(* Logix 5000 AddOnInstructionDefinition export AMCI_MAM; software revision 20.05 *)

TYPE AMCI_Motion_Axis_Output_Data :
STRUCT
   Control_Word_0 : INT;
   Control_Word_1 : INT;
   Position_or_Distance : DINT;
   Programmed_Speed : DINT;
   Acceleration : INT;
   Deceleration : INT;
   Output_Word_8 : INT;
   Output_Word_9 : INT;
END_STRUCT
END_TYPE

TYPE AMCI_Motion_Axis_Input_Data :
STRUCT
   Moving_CW : BOOL;
   Moving_CCW : BOOL;
   In_Hold_State : BOOL;
   Stopped : BOOL;
   At_Home : BOOL;
   Accelerating : BOOL;
   Decelerating : BOOL;
   Move_Complete : BOOL;
   Status_Word_0_Bit_8 : BOOL;
   Status_Word_0_Bit_9 : BOOL;
   Position_Invalid : BOOL;
   Input_Error : BOOL;
   Command_Error : BOOL;
   Configuration_Error : BOOL;
   Module_OK : BOOL;
   Mode_Flag : BOOL;
   IN1_Active : BOOL;
   IN2_Active : BOOL;
   IN3_Active : BOOL;
   IN4_Active : BOOL;
   Status_Word_1_Bit_4 : BOOL;
   Status_Word_1_Bit_5 : BOOL;
   Connection_Was_Lost : BOOL;
   Driver_Fault : BOOL;
   Status_Word_1_Bit_8 : BOOL;
   Invalid_Jog_Change : BOOL;
   Status_Word_1_Bit_10 : BOOL;
   Heartbeat_Bit : BOOL;
   Status_Word_1_Bit_12 : BOOL;
   Status_Word_1_Bit_13 : BOOL;
   Stall_Detected : BOOL;
   Drive_Is_Enabled : BOOL;
   Motor_Position : DINT;
   Encoder_Position : DINT;
   Trapped_Encoder_Position : DINT;
   Input_Word_8 : INT;
   Input_Word_9 : INT;
END_STRUCT
END_TYPE

ADD_ON_INSTRUCTION AMCI_MAM   (* revision 2.0, vendor AMCI, ExecuteEnableInFalse *)
// Absolute and Relative Moves
// Revision note:
// 11/22/22 Initial release of AOI
// 3/6/23 Added logic so that the PC output bit turns on for short moves.  It will also be set for moves of zero steps.
// Help:
// MOTION AXIS MOVE: Performs Absolute or Relative Moves
// AXIS INPUT DATA:  Input data from AMCI motion device.   Uses the AMCI_Motion_Axis_Input_Data User Defined Data Type.
// AXIS OUTPUT DATA; Output data from the AOI to the AMCI motion device.   Uses the AMCI_Motion_Axis_Output_Data User Defined Data Type.
// MOVE TYPE: 0 = Absolute Move, 1 = Relative Move
// POSITION OR DISTANCE: Target Position of the Absolute Move or the distance to move of a Relative                                              Move.
// PROGRAMMED SPEED: Speed of move in units of steps / sec
// ACCELERATION: Acceleration Rate in units of steps / sec / ms
// DECELERATION:  Deceleration Rate in units of steps / sec / ms
// EN (Enable) Set when rung is true, Reset when rung is false
// DN (Done) Set when command is sent to the motion device.  Reset when the rung is false.
// ER (Error) Set when a command or input error failed to clear.  Reset when the rung is false.
// IP (In Process) Set when motion is occurring.   Reset when motion stops or the rung goes false.
// PC (Process Complete) Set when the move is complete.  Reset the next time the rung with the AOI transitions                                       from False to True.
VAR_IN_OUT
   Axis_Input_Data : AMCI_Motion_Axis_Input_Data; {required}
        [0].6   // set when decelerating
   Axis_Output_Data : AMCI_Motion_Axis_Output_Data; {required}
END_VAR
VAR_INPUT
   Type_0_for_standard_1_for_indexed : BOOL;
   Move_type_0_Absolute_1_Relative : BOOL; {required}   // 0=absolute 1=relative
   Position_or_Distance : DINT; {required}
   Programmed_Speed : DINT; {required}
   Acceleration : INT; {required}
   Deceleration : INT; {required}
END_VAR
VAR_OUTPUT
   EN : BOOL; {visible}   // set when rung with AOI is true
   DN : BOOL; {access Read Only, visible}   // set when move was succesfully initiated
   ER : BOOL; {visible}   // set when input error, command error, or configuration error
   IP : BOOL; {visible}   // set when motion occurring
   PC : BOOL; {visible}   // set when process complete
END_VAR
VAR
   command_data_block : INT[10];
        [0]   // Command Bits MSW
        [1]   // Command Bits LSW
        [2]   // Upper Target Position
        [3]   // Lower Target Position
        [4]   // Upper Programmed Speed
        [5]   // Lower Programmed Speed
   motion_occurring : BOOL; {access None}
   Internal_Enable : BOOL; {access None}   // set when driver ready to receive motion command
END_VAR

ROUTINE EnableInFalse   (* ladder *)
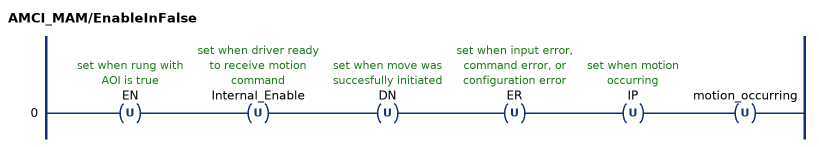
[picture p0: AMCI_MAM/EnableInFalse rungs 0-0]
   0: OTU(EN)OTU(Internal_Enable)OTU(DN)OTU(ER)OTU(IP)OTU(motion_occurring);
END_ROUTINE

ROUTINE Logic   (* ladder *)
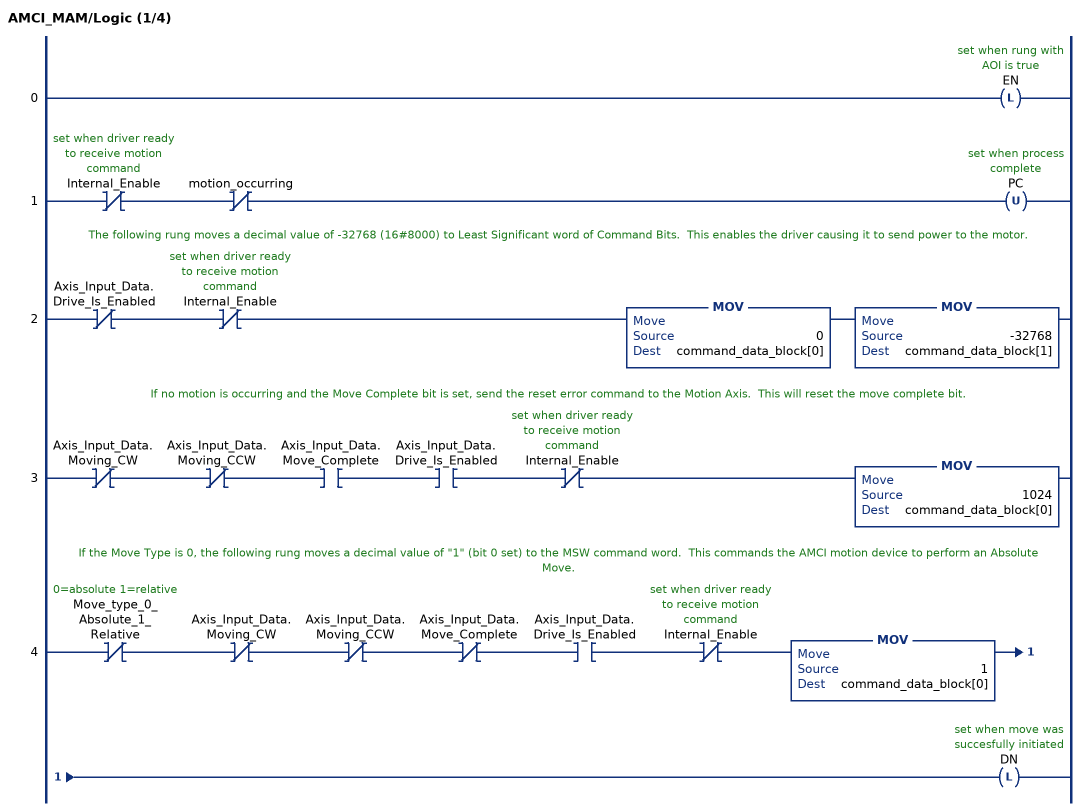
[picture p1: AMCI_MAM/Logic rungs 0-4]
   0: OTL(EN);
   1: XIO(Internal_Enable)XIO(motion_occurring)OTU(PC);
   // The following rung moves a decimal value of -32768 (16#8000) to Least Significant word of Command Bits.  This enables the driver causing it to send power to the motor.
   2: XIO(Axis_Input_Data.Drive_Is_Enabled)XIO(Internal_Enable)MOV(0,command_data_block[0])MOV(-32768,command_data_block[1]);
   // If no motion is occurring and the Move Complete bit is set, send the reset error command to the Motion Axis.  This will reset the move complete bit.
   3: XIO(Axis_Input_Data.Moving_CW)XIO(Axis_Input_Data.Moving_CCW)XIC(Axis_Input_Data.Move_Complete)XIC(Axis_Input_Data.Drive_Is_Enabled)XIO(Internal_Enable)MOV(1024,command_data_block[0]);
   // If the Move Type is 0, the following rung moves a decimal value of "1" (bit 0 set) to the MSW command word.  This commands the AMCI motion device to perform an Absolute Move.
   4: XIO(Move_type_0_Absolute_1_Relative)XIO(Axis_Input_Data.Moving_CW)XIO(Axis_Input_Data.Moving_CCW)XIO(Axis_Input_Data.Move_Complete)XIC(Axis_Input_Data.Drive_Is_Enabled)XIO(Internal_Enable)MOV(1,command_data_block[0])OTL(DN);
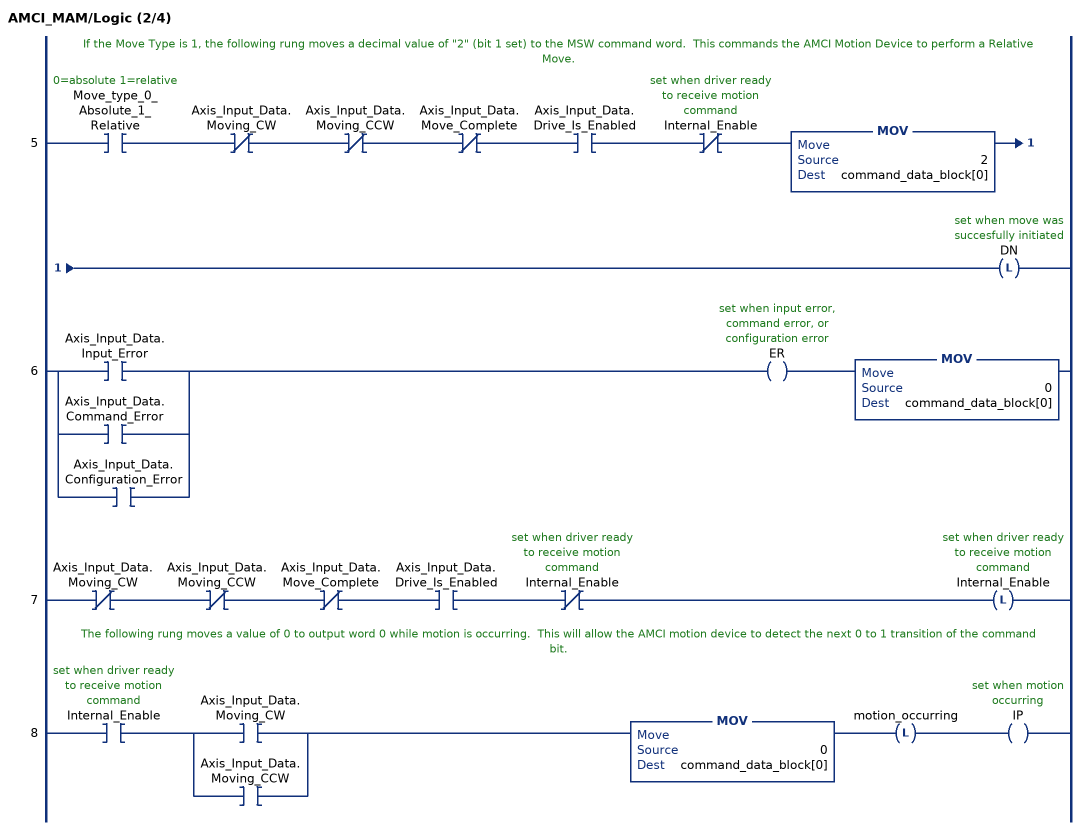
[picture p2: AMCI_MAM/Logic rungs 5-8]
   // If the Move Type is 1, the following rung moves a decimal value of "2" (bit 1 set) to the MSW command word.  This commands the AMCI Motion Device to perform a Relative Move.
   5: XIC(Move_type_0_Absolute_1_Relative)XIO(Axis_Input_Data.Moving_CW)XIO(Axis_Input_Data.Moving_CCW)XIO(Axis_Input_Data.Move_Complete)XIC(Axis_Input_Data.Drive_Is_Enabled)XIO(Internal_Enable)MOV(2,command_data_block[0])OTL(DN);
   6: [XIC(Axis_Input_Data.Input_Error) ,XIC(Axis_Input_Data.Command_Error) ,XIC(Axis_Input_Data.Configuration_Error) ]OTE(ER)MOV(0,command_data_block[0]);
   7: XIO(Axis_Input_Data.Moving_CW)XIO(Axis_Input_Data.Moving_CCW)XIO(Axis_Input_Data.Move_Complete)XIC(Axis_Input_Data.Drive_Is_Enabled)XIO(Internal_Enable)OTL(Internal_Enable);
   // The following rung moves a value of 0 to output word 0 while motion is occurring.  This will allow the AMCI motion device to detect the next 0 to 1 transition of the command bit.
   8: XIC(Internal_Enable)[XIC(Axis_Input_Data.Moving_CW) ,XIC(Axis_Input_Data.Moving_CCW) ]MOV(0,command_data_block[0])OTL(motion_occurring)OTE(IP);
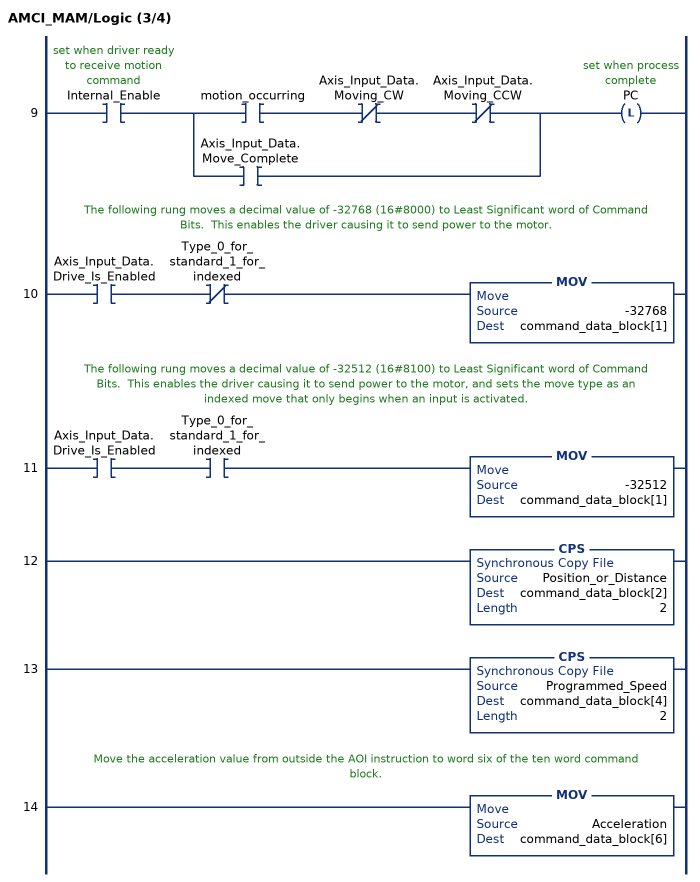
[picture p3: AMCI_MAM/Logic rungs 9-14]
   9: XIC(Internal_Enable)[XIC(motion_occurring) XIO(Axis_Input_Data.Moving_CW) XIO(Axis_Input_Data.Moving_CCW) ,XIC(Axis_Input_Data.Move_Complete) ]OTL(PC);
   // The following rung moves a decimal value of -32768 (16#8000) to Least Significant word of Command Bits.  This enables the driver causing it to send power to the motor.
   10: XIC(Axis_Input_Data.Drive_Is_Enabled)XIO(Type_0_for_standard_1_for_indexed)MOV(-32768,command_data_block[1]);
   // The following rung moves a decimal value of -32512 (16#8100) to Least Significant word of Command Bits.  This enables the driver causing it to send power to the motor, and sets the move type as an indexed move that only begins when an input is activated.
   11: XIC(Axis_Input_Data.Drive_Is_Enabled)XIC(Type_0_for_standard_1_for_indexed)MOV(-32512,command_data_block[1]);
   12: CPS(Position_or_Distance,command_data_block[2],2);
   13: CPS(Programmed_Speed,command_data_block[4],2);
   // Move the acceleration value from outside the AOI instruction to word six of the ten word command block.
   14: MOV(Acceleration,command_data_block[6]);
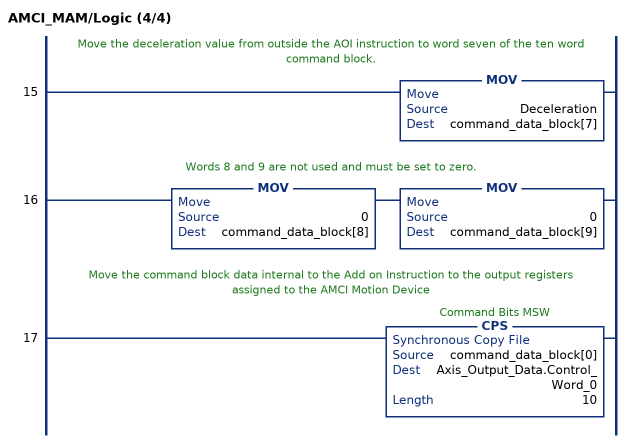
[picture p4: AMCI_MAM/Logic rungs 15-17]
   // Move the deceleration value from outside the AOI instruction to word seven of the ten word command block.
   15: MOV(Deceleration,command_data_block[7]);
   // Words 8 and 9 are not used and must be set to zero.
   16: MOV(0,command_data_block[8])MOV(0,command_data_block[9]);
   // Move the command block data internal to the Add on Instruction to the output registers assigned to the AMCI Motion Device
   17: CPS(command_data_block[0],Axis_Output_Data.Control_Word_0,10);
END_ROUTINE
END_ADD_ON_INSTRUCTION
